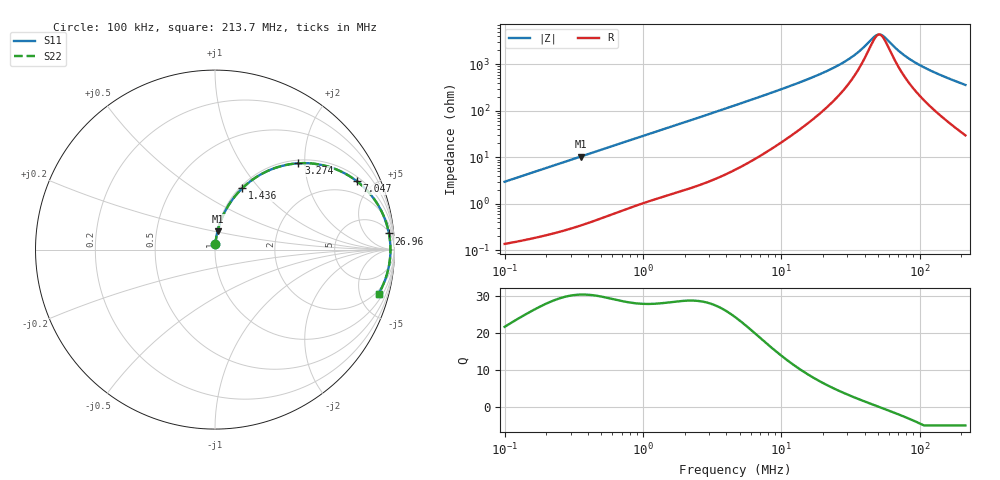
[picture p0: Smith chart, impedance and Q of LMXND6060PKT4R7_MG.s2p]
! LMXND6060PKT4R7_MG  S-PARAMETER MODEL  ( General Type )
! Model Generated by TAIYO YUDEN Corporation (https://www.yuden.co.jp/en/)
! Version 1.0
! TAIYO YUDEN Control No. 191025NI43SB-FBB
! Copyright(c) 2019 TAIYO YUDEN CO.,LTD. All Rights Reserved.
! Product Description (link to TY-COMPAS)
! https://ds.yuden.co.jp/TYCOMPAS/or/detail?pn=LMXND6060PKT4R7MMG&u=M
! Products Name : Inductors
! Characteristics :
!  Inductance : 4.7 uH , SRF(min) : 36 MHz , DC Resistance(max) : 0.108 Ohm
!  Rated Current : Saturation :2000 mA , Temp Rise : 1900 mA (40 degC)
!  Case Size : 6.0 x 6.0 / 0.236 x 0.236 [mm/inch] , Thickness : 1.4 / 0.055 [mm/inch]
!  (Conditions: Temperature = 25 degC , DC Bias Current/Voltage = 0A / 0V)
! External Node Assignments :
!  1  o---GGG---o  2
! GND o---------o GND
! Frequency Range : 0.1MHz  -  213.673535MHz  [ 402 STEP ]
# MHz S RI R 50
! Freq[MHz].  S11 Real  S11 Imag  S21 Real  S21 Imag  S12 Real  S12 Imag  S22 Real  S22 Imag
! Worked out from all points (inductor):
!   401 points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, 100 kHz to 213.7 MHz, reference 50 ohm
!   read as one part in series: L = 4.74 uH near 103.9 kHz
!   highest Q = 30.4 at 354.3 kHz (marker M1), where L = 4.68 uH
!   self-resonance near 50.93 MHz
!   S11 on the Smith chart (normalised r, x): 100 kHz: 1.00, +0.06; 1.436 MHz: 1.03, +0.82; 3.274 MHz: 1.07, +1.86; 7.047 MHz: 1.22, +4.04; 26.96 MHz: 6, +20; 213.7 MHz: 1.59, -7.20
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0.1  0.00227 0.0298  0.9977 -0.0298  0.9977 -0.0298  0.00227 0.0298
0.354331  0.0141 0.1024  0.9859 -0.1024  0.9859 -0.1024  0.0141 0.1024
0.361188  0.0145 0.1043  0.9855 -0.1043  0.9855 -0.1043  0.0145 0.1043
0.762753  0.0534 0.2078  0.9466 -0.2078  0.9466 -0.2078  0.0534 0.2078
1.304567  0.1314 0.3204  0.8686 -0.3204  0.8686 -0.3204  0.1314 0.3204
1.435782  0.1531 0.3427  0.8469 -0.3427  0.8469 -0.3427  0.1531 0.3427
2.10657  0.2712 0.4275  0.7288 -0.4275  0.7288 -0.4275  0.2712 0.4275
3.273683  0.4644 0.481  0.5356 -0.481  0.5356 -0.481  0.4644 0.481
4.71194  0.6368 0.4607  0.3632 -0.4607  0.3632 -0.4607  0.6368 0.4607
7.04712  0.7911 0.3806  0.2089 -0.3806  0.2089 -0.3806  0.7911 0.3806
10.53959  0.8882 0.2796  0.1118 -0.2796  0.1118 -0.2796  0.8882 0.2796
16.69585  0.9446 0.1752  0.0554 -0.1752  0.0554 -0.1752  0.9446 0.1752
26.95988  0.9692 0.0898  0.0308 -0.0898  0.0308 -0.0898  0.9692 0.0898
35.25813  0.9751 0.05  0.0249 -0.05  0.0249 -0.05  0.9751 0.05
48.83978  0.9777 0.00558  0.0223 -0.00558  0.0223 -0.00558  0.9777 0.00558
50.74841  0.9777 0.000464  0.0223 -0.000464  0.0223 -0.000464  0.9777 0.000464
53.75212  0.9777 -0.00721  0.0223 0.00721  0.0223 0.00721  0.9777 -0.00721
60.30341  0.9772 -0.0226  0.0228 0.0226  0.0228 0.0226  0.9772 -0.0226
75.89871  0.9747 -0.0545  0.0253 0.0545  0.0253 0.0545  0.9747 -0.0545
97.37586  0.9691 -0.0918  0.0309 0.0918  0.0309 0.0918  0.9691 -0.0918
140.1569  0.9525 -0.1552  0.0475 0.1552  0.0475 0.1552  0.9525 -0.1552
213.6735  0.9113 -0.246  0.0887 0.246  0.0887 0.246  0.9113 -0.246
